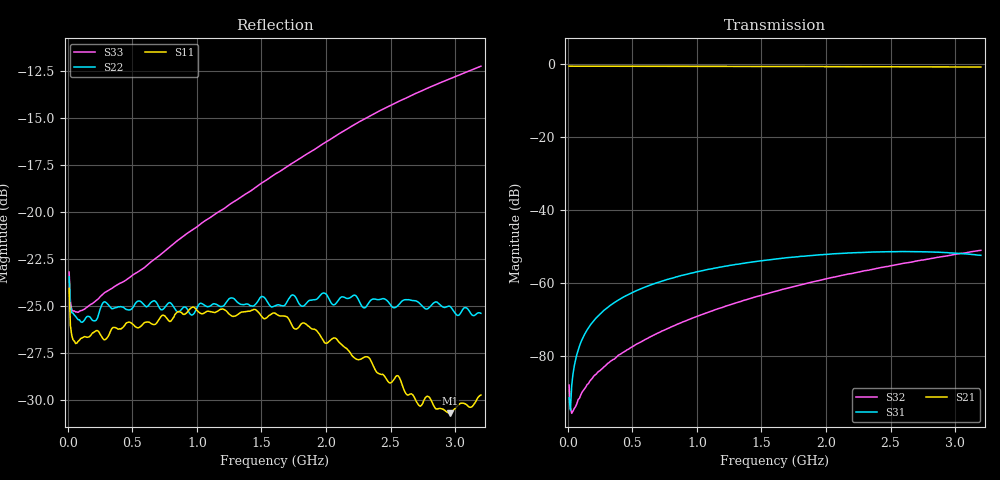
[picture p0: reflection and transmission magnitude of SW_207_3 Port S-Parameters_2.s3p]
! Created _Nov-02-2022_09-58-32
! Type : General
! Retest Level : 0
! Program : FASTESt Rev. 859
! DUT_TempC = 25.0
! Set_V1_Supply_V = 3.0
! V1_Supply_V = 3.0015
! V1_Supply_I = -4e-06
! Set_V2_Supply_V = 0.0
! V2_Supply_V = -0.001
! V2_Supply_I = -5e-06
! RunID = 2
! SN = 1
! Comment = SW-207_SB1_RFc-RF1_room
! Input_Power = 5.0
! Measurement_Comment = None
! Freq	S11db	S11deg	S12db	S12deg	S13db	S13deg	S21db	S21deg	S22db	S22deg	S23db	S23deg	S31db	S31deg	S32db	S32deg	S33db	S33deg
# Hz S dB R 50
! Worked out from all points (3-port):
!   320 points, 10 MHz to 3.2 GHz, reference 50 ohm
!   strongest paths, dB at 10 MHz, 810 MHz, 1.61 GHz, 2.41 GHz, 3.2 GHz:
!     S21: -0.6, -0.6, -0.7, -0.7, -0.8
!     S31: -91.5, -58.8, -53.5, -51.6, -52.5
!     S32: -88.1, -72.0, -62.4, -56.0, -51.1
!   lowest |S11| = -30.7 dB at 2.96 GHz (marker M1), VSWR 1.06, Z = 52.3 + j1.86 ohm
!   |S11| at or under -10 dB: start of sweep to end of sweep
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1e7  -24.06 -41.5  -0.59 1.2  -90.98 -125.3
     -0.59 1.2  -23.44 -38.2  -87.64 -112.1
     -91.55 -125.2  -88.10 -113.7  -23.19 -33.2
6e7  -26.99 -14.8  -0.61 -5.1  -81.22 80.4
     -0.61 -5.1  -25.55 -13.3  -94.11 -90.0
     -81.18 80.1  -93.98 -92.1  -25.31 -7.6
1.6e8  -26.65 -17.7  -0.61 -14.2  -72.39 73.9
       -0.61 -14.2  -25.55 -16.7  -87.56 -114.9
       -72.36 73.9  -87.68 -114.8  -25.00 -3.7
3.2e8  -26.51 -28.4  -0.62 -28.4  -66.48 61.6
       -0.62 -28.4  -24.98 -27.6  -81.98 -140.4
       -66.45 61.6  -81.90 -139.7  -24.14 -5.2
8.5e8  -25.31 -85.8  -0.64 -74.7  -58.33 19.1
       -0.64 -74.8  -25.31 -83.8  -71.43 154.2
       -58.35 19.1  -71.36 154.5  -21.51 -29.6
1.21e9  -25.18 -127.1  -0.66 -106.2  -55.56 -10.2
        -0.65 -106.2  -24.97 -124.0  -66.65 116.8
        -55.54 -10.2  -66.60 117.1  -19.81 -54.3
1.61e9  -25.39 -167.0  -0.69 -141.0  -53.51 -42.5
        -0.68 -141.1  -24.97 -162.0  -62.41 79.5
        -53.51 -42.8  -62.37 79.7  -17.96 -86.2
2.24e9  -27.84 128.9  -0.73 164.1  -51.77 -94.1
        -0.73 164.0  -24.52 145.4  -57.20 25.2
        -51.75 -94.4  -57.18 25.4  -15.26 -138.8
2.96e9  -30.71 37.6  -0.80 101.3  -51.82 -152.3
        -0.80 101.2  -25.01 82.1  -52.51 -31.2
        -51.84 -152.5  -52.51 -31.3  -12.90 160.5
3.2e9  -29.73 0.4  -0.83 80.3  -52.52 -170.4
       -0.82 80.2  -25.38 56.0  -51.11 -49.2
       -52.48 -170.7  -51.11 -49.3  -12.23 139.7
